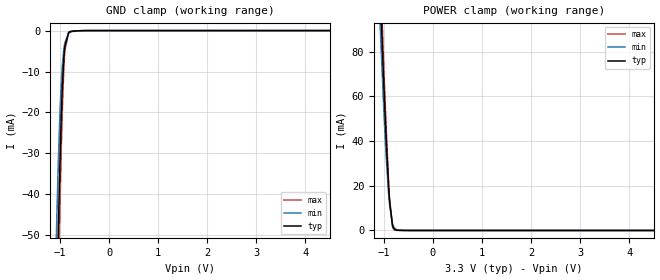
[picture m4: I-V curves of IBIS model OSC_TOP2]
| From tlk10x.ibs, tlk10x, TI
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|   Model
[Model]   OSC_TOP2
Model_type   Input
Vinl = 0.99
Vinh = 2.31
|   typ   min   max
C_comp   0.431pF   0.350pF   0.515pF
[Voltage Range]   3.3   3   3.6
[Temperature Range]   25   125   -40
[Power Clamp Reference]   3.3   3   3.6
[GND Clamp Reference]   -0   -0   -0
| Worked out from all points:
|   GND clamp passes 1 mA (typ) near -0.84 V on its own axis
|   POWER clamp passes 1 mA (typ) near -0.80 V on its own axis
[GND Clamp]
|   Voltage   I(typ)   I(min)   I(max)
-3.3V     -1.746A    -1.721A    -1.773A
-1.102V   -87.09mA   -63.73mA   -104.4mA
-1.073V   -69.09mA   -48.49mA   -84.87mA
-1.043V   -52.2mA    -34.96mA   -66.12mA
-1.033V   -46.89mA   -30.9mA    -60.09mA
-1.003V   -32.2mA    -20.31mA   -42.91mA
-973.5mV  -19.93mA   -12.33mA   -27.6mA
-953.7mV  -13.46mA   -8.474mA   -18.91mA
-924mV    -6.648mA   -4.605mA   -9.048mA
-904.2mV  -3.895mA   -3.016mA   -4.901mA
-805.2mV  -325.1uA   -465.7uA   -276.1uA
6.59V     0A         0A         0A
[POWER Clamp]
|   Voltage   I(typ)   I(min)   I(max)
-3.3V     1.589A     1.523A     1.646A
-1.082V   111.3mA    95.44mA    122.8mA
-1.003V   66.42mA    55.28mA    74.51mA
-973.5mV  50.89mA    41.87mA    57.46mA
-953.7mV  41.14mA    33.68mA    46.6mA
-904.2mV  20.02mA    16.72mA    22.37mA
-884.4mV  13.46mA    11.71mA    14.56mA
-825mV    2.514mA    3.119mA    1.881mA
-775.5mV  457.5uA    926.3uA    236.1uA
-696.3mV  60.44uA    199.1uA    56.09uA
-478.5mV  3.327uA    9.453uA    3.221uA
6.59V     0A         0A         0A
